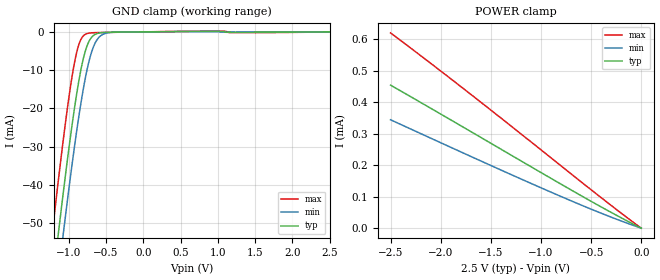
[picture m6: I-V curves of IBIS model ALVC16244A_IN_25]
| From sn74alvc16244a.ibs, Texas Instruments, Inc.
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[Model]   ALVC16244A_IN_25
Model_type  Input
Vinl=0.7
Vinh=1.7
| variable   typ   min   max
C_comp   0.95pF   0.63pF   1.22pF
[Temperature Range]   40   100   -40
| Ambient temperature   25   85   -40
[Voltage range]   2.5   2.3   2.7
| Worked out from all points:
|   GND clamp passes 1 mA (typ) near -0.67 V on its own axis
[GND Clamp]
| ALVC16244A_IN_25
|   Voltage   I(typ)   I(min)   I(max)
-2.5V     -300.5mA   -309.8mA   -289mA
-1.22V    -66.17mA   -76.96mA   -52.33mA
-1.15V    -54.43mA   -65.24mA   -40.55mA
-1.125V   -50.33mA   -61.12mA   -36.45mA
-1.07V    -41.49mA   -52.23mA   -27.72mA
-980mV    -27.83mA   -38.28mA   -14.76mA
-910mV    -18.27mA   -28.18mA   -6.803mA
-845mV    -10.75mA   -19.66mA   -2.328mA
-770mV    -4.556mA   -11.37mA   -576.1uA
-645mV    -651.1uA   -2.896mA   -208.6uA
-485mV    -118.7uA   -297.1uA   -147.3uA
2.5V      1.114nA    22.86uA    -45.09uA
[POWER Clamp]
| ALVC16244A_IN_25
|   Voltage   I(typ)   I(min)   I(max)
-2.5V     453.8uA    343.9uA    619.5uA
-1.745V   314.9uA    234.2uA    435.8uA
-845mV    147.9uA    106.7uA    209.1uA
-375mV    63.11uA    44.35uA    90.67uA
-31.15fV  1.114nA    59.61nA    7.183pA
